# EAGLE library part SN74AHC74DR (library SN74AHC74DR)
Dual Positive-Edge-Triggered D-Type Flip-Flops With Clear and Preset Source: Datasheet
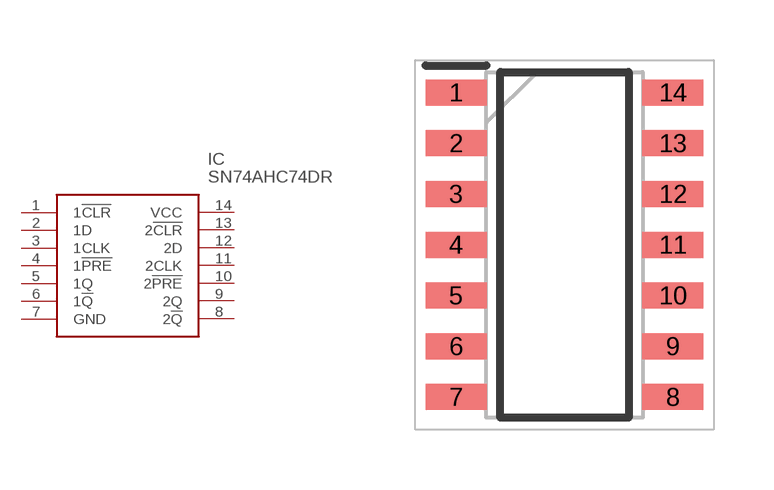
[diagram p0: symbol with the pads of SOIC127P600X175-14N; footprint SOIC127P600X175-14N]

Designator prefix IC

## SN74AHC74DR (Description: Dual Positive-Edge-Triggered D-Type Flip-Flops With Clear and Preset; Height: 1.75mm; Manufacturer_Name: Texas Instruments; Manufacturer_Part_Number: SN74AHC74DR; Mouser_Part_Number: 595-SN74AHC74DR; Mouser_Price-Stock: https://www.mouser.co.uk/ProductDetail/Texas-Instruments/SN74AHC74DR?qs=st7IWvlL5%2FgP9OJq63EsFQ%3D%3D)  [SOIC127P600X175-14N]
1  1!CLR
2  1D
3  1CLK
4  1!PRE
5  1Q
6  1!Q
7  GND
8  2!Q
9  2Q
10  2!PRE
11  2CLK
12  2D
13  2!CLR
14  VCC

## Footprint SOIC127P600X175-14N (pad centres in mm)
D (-R-PDSO-G14)
smd 1.525 x 0.65: 1 -2.712,3.81; 2 -2.712,2.54; 3 -2.712,1.27; 4 -2.712,0; 5 -2.712,-1.27; 6 -2.712,-2.54; 7 -2.712,-3.81; 8 2.712,-3.81; 9 2.712,-2.54; 10 2.712,-1.27; 11 2.712,0; 12 2.712,1.27; 13 2.712,2.54; 14 2.712,3.81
